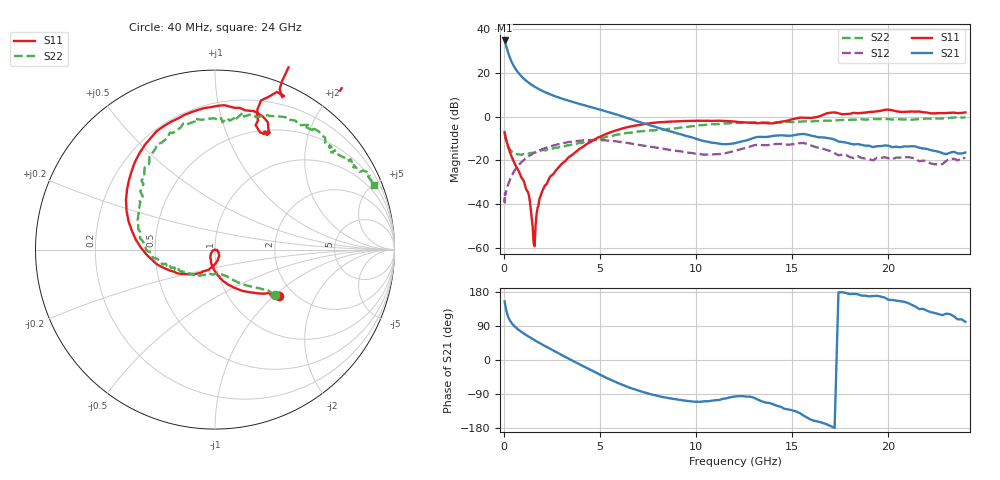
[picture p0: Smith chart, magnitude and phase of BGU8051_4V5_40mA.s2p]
! BGU8051_4V5_40mA
! Date/time Tue Jun 16 11:03:17 2015
! VAR V_out= 4.5000
! VAR I_out= 40.0100
! VAR V_in= 4.6280
! VAR I_in= 0.5372
# MHz S MA R 50
!  Freq-MHz  S11-mag  S11-arg  S21-mag  S21-arg  S12-mag  S12-arg  S22-mag  S22-arg
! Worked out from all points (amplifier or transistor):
!   187 points, 40 MHz to 24 GHz, reference 50 ohm
!   highest |S21| = 34.8 dB at 40 MHz (marker M1)
!   |S21| within 3 dB of that: start of sweep to 137.7 MHz
!   unconditionally stable (mu >= 1): 485.1 MHz to 14.05 GHz
!   at 750 MHz: K = 1.01, MAG = 20.5 dB, |S12| = -22.4 dB
!   at 5.4 GHz: K = 1.20, MAG = 3.9 dB, |S12| = -11.0 dB
!   at 24 GHz: K = -0.79, MSG = 1.3 dB, |S12| = -19.0 dB
!   lowest NFmin = 0.33 dB at 400 MHz
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40  0.4412 -35.7  55.16 154.7  0.01432 31.6  0.4187 -37.4
60  0.3881 -38.5  51.91 149.1  0.01786 55.5  0.3656 -37.4
80  0.3572 -43.3  47.96 143.3  0.01646 38.6  0.3304 -40.8
120  0.2996 -52.0  41.6 132.8  0.01909 44.7  0.2818 -46.3
160  0.2557 -59.8  35.9 124.4  0.02251 48.8  0.2491 -50.9
220  0.2065 -69.9  29.29 114.8  0.02762 53.7  0.2142 -56.2
280  0.1703 -77.2  24.37 107.7  0.03273 56.5  0.1897 -61.1
360  0.1354 -86.0  19.77 100.7  0.04005 59.5  0.1662 -65.2
440  0.11 -93.1  16.56 95.2  0.04729 60.5  0.1544 -70.2
550  0.08669 -102.1  13.52 89.1  0.05745 60.7  0.1419 -75.0
750  0.0589 -113.7  10.08 80.3  0.0757 59.1  0.1366 -83.4
950  0.03857 -129.5  8.031 72.8  0.0937 56.4  0.1339 -90.3
1300  0.01588 -157.7  5.914 61.4  0.1241 50.3  0.1431 -102.0
1550  0.001266 164.7  4.978 53.7  0.1448 45.3  0.1487 -110.3
1850  0.0131 -10.1  4.181 45.0  0.1683 39.1  0.1598 -118.1
2600  0.04983 -68.6  2.983 24.2  0.2199 22.8  0.1901 -133.6
4100  0.2012 -136.6  1.855 -15.7  0.2836 -10.7  0.2502 -156.0
8200  0.7457 112.2  0.5246 -97.3  0.1855 -76.5  0.4985 147.4
12200  0.7492 66.7  0.2574 -95.4  0.1728 -73.8  0.7142 103.3
16200  0.9631 68.0  0.349 -160.9  0.2012 -149.7  0.7891 70.6
20200  1.389 34.2  0.1997 158.4  0.1043 -158.2  0.8546 44.0
24000  1.249 21.3  0.15 100.7  0.1116 -176.3  0.9581 22.0
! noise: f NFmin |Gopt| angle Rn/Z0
400  0.331  0.1298  21.7  0.0551
550  0.3393  0.09895  33.62  0.0531
950  0.3732  0.0642  94.88  0.0489
1250  0.4099  0.08635  133.1  0.0468
1600  0.4648  0.1224  153.6  0.0457
1900  0.5223  0.1498  163.9  0.0459
2250  0.6016  0.1763  173.3  0.0476
2600  0.6939  0.1982  181.7  0.0511
3300  0.9179  0.237  197.2  0.0639
4000  1.194  0.2814  210.5  0.0853
